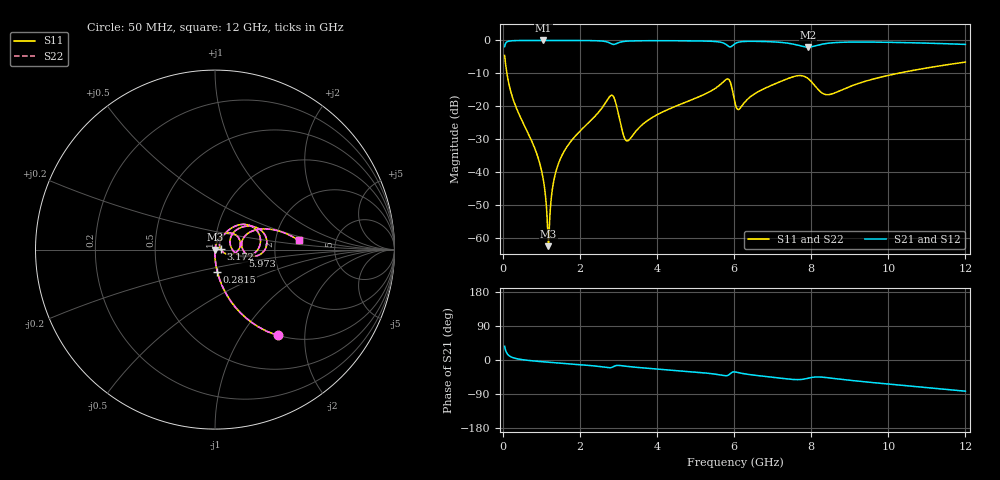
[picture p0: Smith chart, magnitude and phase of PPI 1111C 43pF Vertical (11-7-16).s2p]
# GHz S MA R 50
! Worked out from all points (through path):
!   1601 points, 50 MHz to 12 GHz, reference 50 ohm
!   highest |S21| = -0.01 dB at 1.058 GHz (marker M1); lowest = -2.0 dB at 7.915 GHz (marker M2)
!   group delay of S21, straight-line fit = 18.8 ps
!   lowest |S11| = -62.4 dB at 1.185 GHz (marker M3), VSWR 1.00, Z = 50.1 - j0.014 ohm
!   |S11| at or under -10 dB: 109.5 MHz to 10.24 GHz (10.13 GHz wide, 196 % of centre)
!   |S22| runs from -62.4 to -4.6 dB; largest |S21 - S12| = 0
!   S11 on the Smith chart (normalised r, x): 50 MHz: 0.99, -1.46; 281.5 MHz: 0.99, -0.25; 3.172 GHz: 1.07, +0.00; 5.973 GHz: 1.36, -0.10; 12 GHz: 2.72, +0.35
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0.05  0.5919 -53.9  0.8058 36.0  0.8058 36.0  0.5919 -53.9
0.2815313  0.1227 -84.2  0.992 5.7  0.992 5.7  0.1227 -84.2
0.856625  0.02113 -91.3  0.9991 -3.0  0.9991 -3.0  0.02113 -91.3
1.058281  0.007447 -89.4  0.9992 -4.8  0.9992 -4.8  0.007447 -89.4
1.18525  0.0007556 -10.7  0.9992 -5.9  0.9992 -5.9  0.0007556 -10.7
1.222594  0.002122 62.6  0.9992 -6.2  0.9992 -6.2  0.002122 62.6
1.319687  0.007146 76.5  0.9991 -6.9  0.9991 -6.9  0.007146 76.5
1.446656  0.01354 78.3  0.9989 -7.9  0.9989 -7.9  0.01354 78.3
2.044156  0.04433 74.8  0.9969 -12.6  0.9969 -12.6  0.04433 74.8
2.828375  0.1475 21.7  0.884 -19.5  0.884 -19.5  0.1475 21.7
3.171937  0.03192 3.1  0.9696 -16.2  0.9696 -16.2  0.03192 3.1
4.038312  0.07634 61.0  0.9904 -24.1  0.9904 -24.1  0.07634 61.0
5.808406  0.2587 22.1  0.8571 -41.4  0.8571 -41.4  0.2587 22.1
5.972719  0.1589 -13.5  0.8474 -31.6  0.8474 -31.6  0.1589 -13.5
6.025  0.1126 -8.8  0.8948 -31.5  0.8948 -31.5  0.1126 -8.8
6.137031  0.09102 22.8  0.9467 -33.9  0.9467 -33.9  0.09102 22.8
7.130375  0.2283 35.1  0.9424 -47.1  0.9424 -47.1  0.2283 35.1
7.914594  0.2655 -3.6  0.7928 -48.2  0.7928 -48.2  0.2655 -3.6
8.019156  0.2321 -8.8  0.8048 -46.0  0.8048 -46.0  0.2321 -8.8
8.452344  0.1505 9.5  0.9086 -47.0  0.9086 -47.0  0.1505 9.5
10.01331  0.2961 22.9  0.9366 -63.6  0.9366 -63.6  0.2961 22.9
12  0.4693 6.2  0.8703 -82.3  0.8703 -82.3  0.4693 6.2
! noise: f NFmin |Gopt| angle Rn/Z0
0.05  0.0003317  0.8514  0.7951  0.0004757
1.372  0.00336  0.6427  6.719  0.001772
2.701  0.03307  0.9173  13.25  0.08706
4.031  0.01566  0.7634  19.51  0.01306
5.36  0.02452  0.7987  25.68  0.024
6.682  0.03363  0.819  31.77  0.03603
8.012  0.1255  0.9396  37.86  0.4149
9.341  0.04686  0.8274  43.32  0.04942
10.67  0.0373  0.7684  48.28  0.0274
12  0.03634  0.7459  52.96  0.02315
